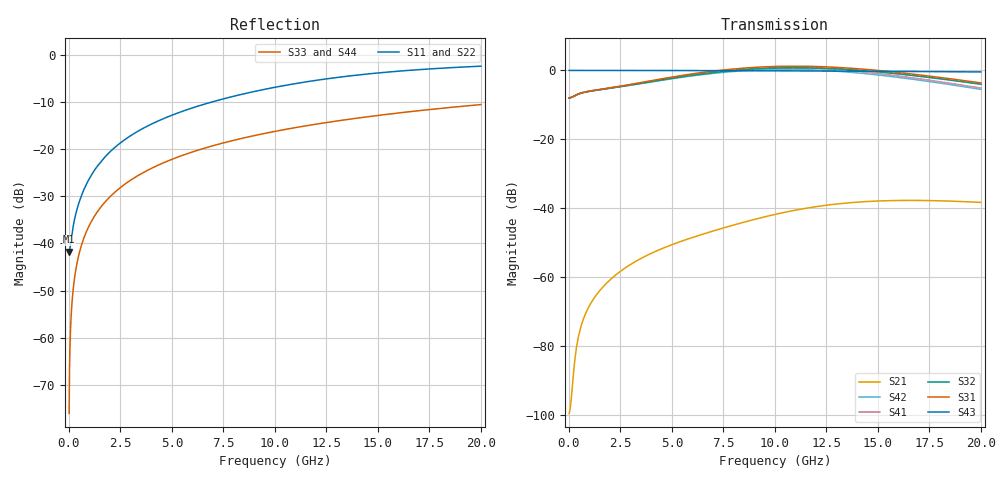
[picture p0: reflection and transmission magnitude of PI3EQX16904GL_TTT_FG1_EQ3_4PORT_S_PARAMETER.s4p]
! NPort=4 DATA=2000 NOISE=0 GROUPDELAY=0 COMPLEX_DATAFORMAT=POLAR
! NumOfBlock=1 NumOfParam=0
! .MODEL Smodel S TSTONEFILE=PI3EQX16904GL_TTT_FG1_EQ3_4PORT_S_PARAMETER.s4p TYPE=S
!  -- The above .MODEL line can be used for the S element in the netlist.
! The s parameter is extracted from the linear redriver, it is not bi-directional; only s(4,1)s(4,2) and s(3,1)s(3,2)
! should be the insertion loss
!Port definition:
!Port1 = input+
!Port2 = input-
!Port3 = output+
!Port4 = output-
# Hz S MA R  50
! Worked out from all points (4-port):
!   2000 points, 10 MHz to 20 GHz, reference 50 ohm
!   strongest paths, dB at 10 MHz, 5.01 GHz, 10.01 GHz, 15.01 GHz, 20 GHz:
!     S43: 0.0, 0.0, -0.1, -0.3, -0.4
!     S31: -8.0, -1.9, 1.1, 0.0, -3.6
!     S32: -8.0, -2.3, 0.7, -0.4, -4.0
!     S41: -8.0, -2.0, 0.7, -0.9, -5.1
!     S42: -8.0, -2.4, 0.3, -1.3, -5.5
!     S21: -99.6, -50.6, -41.8, -37.9, -38.3
!   lowest |S11| = -41.7 dB at 10 MHz (marker M1), VSWR 1.02, Z = 49.2 - j0.0603 ohm
!   |S11| at or under -10 dB: start of sweep to 6.903 GHz
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1e7  0.008182 -175.7  1.05e-05 7.6  0 0.0  0 0.0
     1.05e-05 7.6  0.008182 -175.7  0 0.0  0 0.0
     0.3995 0.2  0.3995 -179.8  0.0001571 -90.0  1 -0.0
     0.3995 -179.8  0.3995 0.2  1 -0.0  0.0001571 -90.0
2e8  0.01483 -130.6  3.387e-05 105.9  0 0.0  0 0.0
     3.387e-05 105.9  0.01483 -130.6  0 0.0  0 0.0
     0.4168 4.9  0.4166 -175.3  0.003142 -90.2  1 -0.2
     0.4168 -175.5  0.4166 4.3  1 -0.2  0.003142 -90.2
6.2e8  0.03268 -112.4  0.0002073 113.9  0 0.0  0 0.0
       0.0002073 113.9  0.03268 -112.4  0 0.0  0 0.0
       0.4722 5.5  0.4712 -175.0  0.009738 -90.6  0.9999 -0.6
       0.4721 -175.6  0.4711 3.9  0.9999 -0.6  0.009738 -90.6
2.97e9  0.1383 -101.6  0.001509 98.3  0 0.0  0 0.0
        0.001508 98.2  0.1383 -101.6  0 0.0  0 0.0
        0.6237 -7.2  0.6115 171.1  0.0466 -92.8  0.9988 -2.7
        0.6209 167.5  0.6087 -14.2  0.9988 -2.7  0.0466 -92.8
1.026e10  0.4669 -113.5  0.00853 53.6  0 0.0  0 0.0
          0.008435 54.2  0.466 -113.5  0 0.0  0 0.0
          1.147 -99.8  1.089 80.0  0.1589 -99.5  0.9863 -9.1
          1.089 62.4  1.034 -117.9  0.9863 -9.1  0.1589 -99.5
1.441e10  0.6281 -123.8  0.01255 12.9  0 0.0  0 0.0
          0.01245 14.0  0.6268 -123.7  0 0.0  0 0.0
          1.035 -163.9  0.9872 16.2  0.2203 -103.2  0.9734 -12.7
          0.9401 -8.2  0.8963 171.9  0.9734 -12.7  0.2203 -103.2
2e10  0.7637 -135.9  0.01217 -33.5  0 0.0  0 0.0
      0.01213 -32.0  0.7631 -135.8  0 0.0  0 0.0
      0.6587 121.5  0.6302 -58.3  0.2986 -108.1  0.9506 -17.4
      0.5547 -90.5  0.5306 89.8  0.9506 -17.4  0.2986 -108.1
